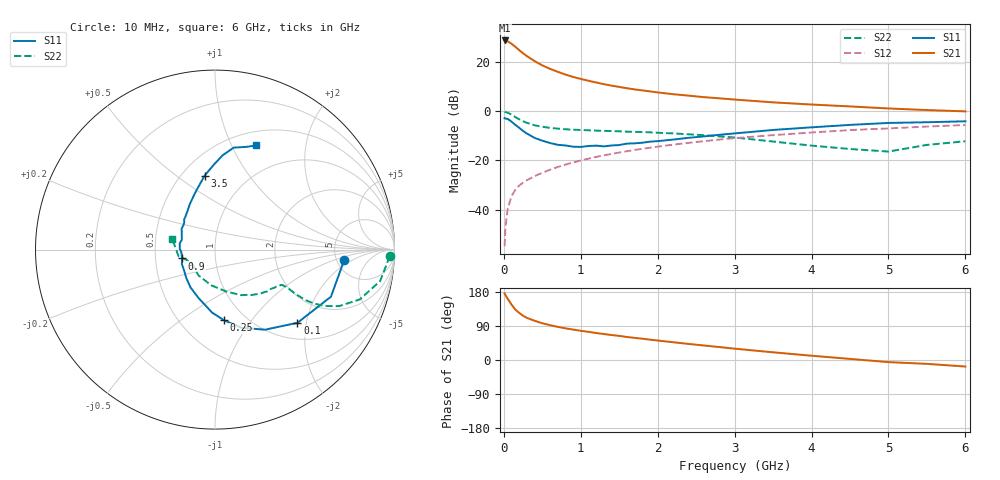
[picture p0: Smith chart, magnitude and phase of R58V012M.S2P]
! SIEMENS Small Signal Semiconductors
! BFR183
! Si NPN RF Bipolar Junction Transistor in SOT23
! VCE = 8 V  IC = 12 mA
! Common Emitter S-Parameters:  May  1996
# GHz  S  MA  R  50
!  f  S11  S21  S12  S22
! GHz  MAG  ANG  MAG  ANG  MAG  ANG  MAG  ANG
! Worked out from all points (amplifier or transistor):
!   36 points, 10 MHz to 6 GHz, reference 50 ohm
!   highest |S21| = 28.8 dB at 10 MHz (marker M1)
!   |S21| within 3 dB of that: start of sweep to 164.7 MHz
!   unconditionally stable (mu >= 1): 773.6 MHz to 2.616 GHz
!   at 250 MHz: K = 0.66, MSG = 26.3 dB, |S12| = -29.0 dB
!   at 1.4 GHz: K = 1.05, MAG = 12.6 dB, |S12| = -17.4 dB
!   at 6 GHz: K = 0.89, MSG = 2.8 dB, |S12| = -5.6 dB
!   S11 on the Smith chart (normalised r, x): 10 MHz: 5.86, -1.35; 100 MHz: 1.36, -1.78; 250 MHz: 0.80, -0.75; 900 MHz: 0.69, -0.07; 3.5 GHz: 0.64, +0.64; 6 GHz: 0.66, +1.25
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0.01  0.7216 -4.4  27.49 175.7  0.0018 84.3  0.9736 -2.1
0.02  0.7101 -8.8  27.39 171.8  0.0042 84.7  0.9624 -4.4
0.05  0.6973 -22.1  26.41 161.5  0.0103 80.3  0.9365 -10.8
0.1  0.6143 -41.6  23.55 146.2  0.0188 72.9  0.853 -19.0
0.15  0.5261 -58.0  20.36 133.0  0.0253 67.7  0.7597 -24.5
0.2  0.4607 -71.1  17.46 124.2  0.0307 65.0  0.6854 -27.3
0.25  0.3975 -82.6  15.07 116.8  0.0353 63.8  0.6255 -28.6
0.3  0.3515 -92.6  13.21 111.2  0.0395 64.6  0.5795 -29.1
0.4  0.2863 -108.3  10.46 103.5  0.0479 64.9  0.5186 -28.9
0.5  0.2515 -122.7  8.553 96.9  0.0559 65.4  0.4823 -28.3
0.6  0.2258 -134.9  7.288 91.9  0.0646 66.4  0.4592 -27.8
0.7  0.2073 -146.5  6.335 87.5  0.0732 67.0  0.4428 -27.7
0.9  0.1899 -165.0  4.987 80.3  0.0907 66.9  0.4209 -27.9
1.1  0.1963 178.7  4.162 74.3  0.1084 66.2  0.4095 -29.4
1.3  0.1928 163.3  3.554 68.5  0.1265 65.2  0.3988 -31.0
1.6  0.2196 147.8  2.933 60.7  0.1536 63.2  0.3835 -34.5
2.2  0.2647 125.3  2.22 46.9  0.2089 58.1  0.354 -43.5
3.5  0.4159 98.0  1.514 20.3  0.326 43.1  0.2418 -75.0
4.5  0.527 85.4  1.252 2.9  0.4132 31.1  0.1705 -122.8
5  0.5778 79.6  1.138 -5.6  0.4471 23.8  0.1511 -153.0
5.5  0.5968 73.4  1.056 -10.2  0.4878 19.6  0.2064 -169.6
6  0.6241 68.4  0.993 -17.2  0.5237 12.2  0.2452 166.1
